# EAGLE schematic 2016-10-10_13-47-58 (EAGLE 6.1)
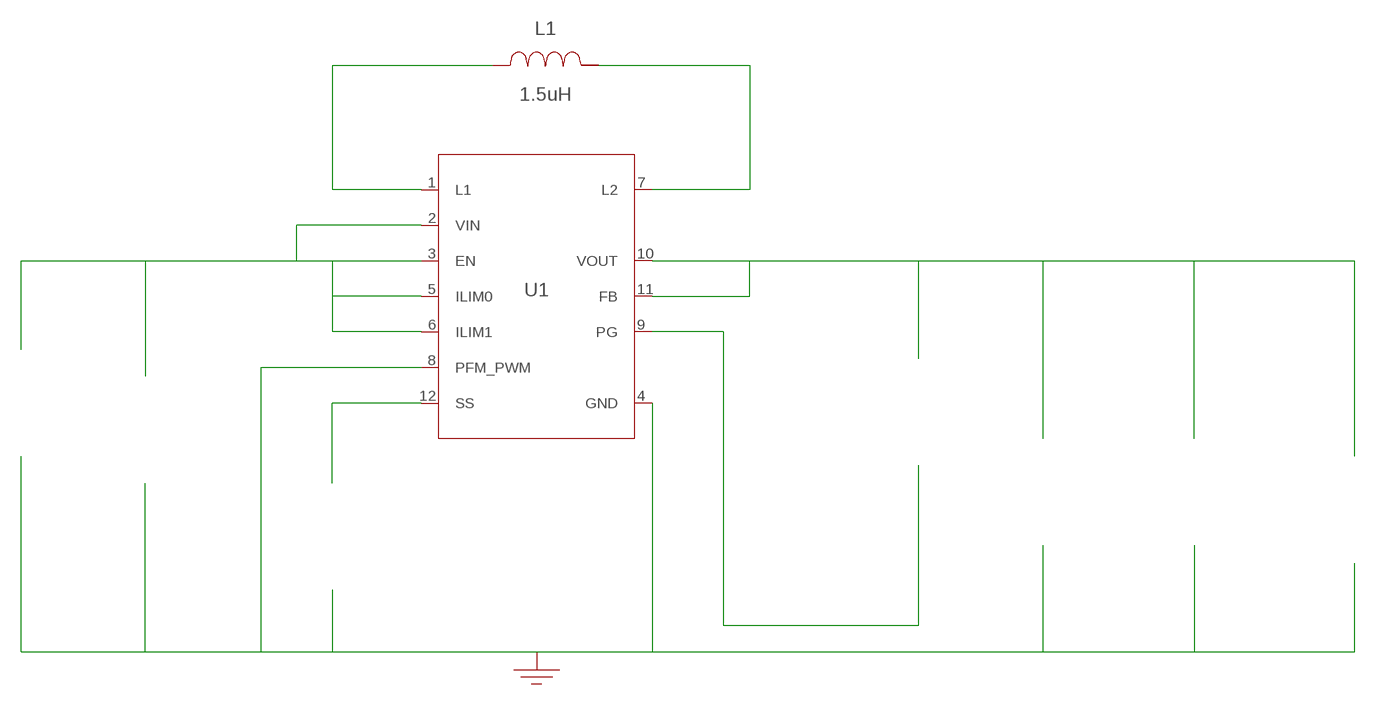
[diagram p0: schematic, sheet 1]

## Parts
CIN  10uF  LMK107BBJ106MAHTLMK107BBJ106MAHT  [0603]  (not placed on a sheet)
COUT  10uF  CL10A106MQ8NNNCCL10A106MQ8NNNC  [0603]  (not placed on a sheet)
COUTX  10uF  CL10A106MQ8NNNCCL10A106MQ8NNNC  [0603]  (not placed on a sheet)
CSS  1nF  GRM155R61A102KA01DGRM155R61A102KA01D  [0402]  (not placed on a sheet)
GND  WB_GND  WB_GNDWB_GND  [WB_GND]
IOUT  WB_CURRENT_LOAD  WB_CURRENT_LOADWB_CURRENT_LOAD  [WB_CURRENT_LOAD]  (not placed on a sheet)
L1  1.5uH  LQM2HPN1R5MG0LLQM2HPN1R5MG0L  [1008]
RPG  100k  CRCW0603100KFKEACRCW0603100KFKEA  [0603]  (not placed on a sheet)
U1  TPS63051YFFR  TPS63051YFFRTPS63051YFFR  [YFF0012AFAF]
VIN  WB_BATTERY  WB_BATTERYWB_BATTERY  [WB_BATTERY]  (not placed on a sheet)

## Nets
0: Cin.2@2 Cout.2@2 Coutx.2@2 Css.2@2 GND.1 Iout.-@2 U1.4(GND) U1.8(PFM_PWM) Vin.-@2
2: Cin.1@1 U1.2(VIN) U1.3(EN) U1.5(ILIM0) U1.6(ILIM1) Vin.+@1
3: Css.1@1 U1.12(SS)
4: Cout.1@1 Coutx.1@1 Iout.+@1 Rpg.1@1 U1.10(VOUT) U1.11(FB)
5: L1.1 U1.1(L1)
6: L1.2 U1.7(L2)
8: Rpg.2@2 U1.9(PG)
Unconnected: CIN.1 CIN.2 COUT.1 COUT.2 COUTX.1 COUTX.2 CSS.1 CSS.2 IOUT.1(+) IOUT.2(-) RPG.1 RPG.2 VIN.1(+) VIN.2(-)

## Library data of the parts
CIN = AcceleratedDesigns_Lib:LMK107BBJ106MAHT; Cap: 1.0E-5; ESR: 0; IRMS: 0; Manufacturer_Name: Taiyo Yuden; Manufacturer_Part_Number: LMK107BBJ106MAHT; VDC: 10; Vendor: Taiyo Yuden
COUT COUTX = AcceleratedDesigns_Lib:CL10A106MQ8NNNC; Cap: 1.0E-5; ESR: 0; IRMS: 0; Manufacturer_Name: Samsung Electro-Mechanics; Manufacturer_Part_Number: CL10A106MQ8NNNC; VDC: 6.3; Vendor: Samsung Semiconductor
CSS = AcceleratedDesigns_Lib:GRM155R61A102KA01D; Cap: 1.0E-9; ESR: 0.0; IRMS: 0.0; Manufacturer_Name: MuRata; Manufacturer_Part_Number: GRM155R61A102KA01D; VDC: 10.0; Vendor: MuRata
GND = AcceleratedDesigns_Lib:WB_GND; Manufacturer_Name: WB_GND; Manufacturer_Part_Number: WB_GND; PowerPortType: POWER_GROUND; Value: Value
IOUT = AcceleratedDesigns_Lib:WB_CURRENT_LOAD; Manufacturer_Name: WB_CURRENT_LOAD; Manufacturer_Part_Number: WB_CURRENT_LOAD; PowerPortType: POWER_GROUND; Value: Value
L1 = AcceleratedDesigns_Lib:LQM2HPN1R5MG0L; DCR: 0.07; IDC: 1.5; L: 1.5E-6; Manufacturer_Name: MuRata; Manufacturer_Part_Number: LQM2HPN1R5MG0L; Vendor: MuRata
RPG = AcceleratedDesigns_Lib:CRCW0603100KFKEA; Manufacturer_Name: Vishay-Dale; Manufacturer_Part_Number: CRCW0603100KFKEA; Power: 0.1; Resistance: 100000.0; Tolerance: 1.0; Vendor: Vishay-Dale
U1 = AcceleratedDesigns_Lib:TPS63051YFFR; Datasheet_URL: http://www.ti.com/product/TPS63051; Frequency: 2500000.0; Imax: 1.0; Manufacturer_Name: Texas Instruments; Manufacturer_Part_Number: TPS63051YFFR; Mktg_Package: RMW0012A; NSID: TPS63051RMWR; Package: RMW0012A; Vendor: Texas Instruments
VIN = AcceleratedDesigns_Lib:WB_BATTERY; Manufacturer_Name: WB_BATTERY; Manufacturer_Part_Number: WB_BATTERY; PowerPortType: POWER_GROUND; Value: Value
